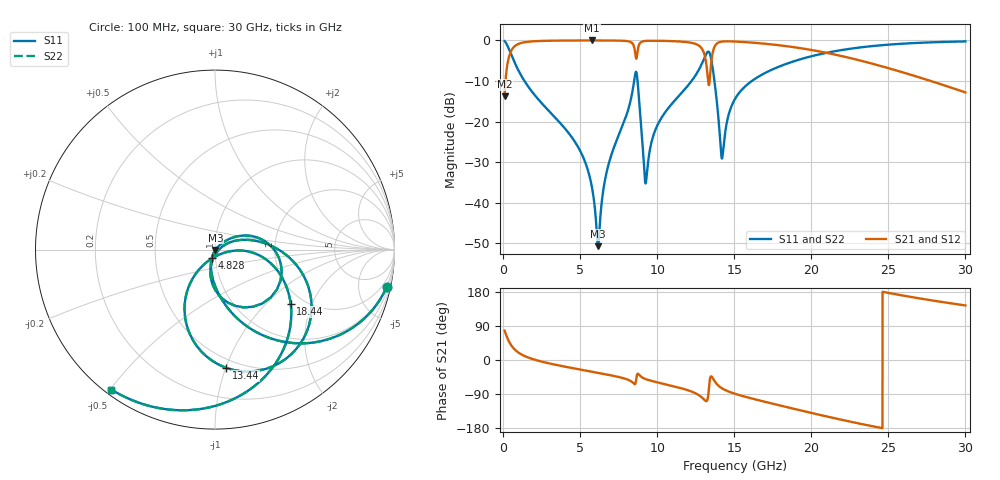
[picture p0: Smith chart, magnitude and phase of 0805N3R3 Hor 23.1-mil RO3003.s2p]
# GHz S MA R 50
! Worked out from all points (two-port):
!   3201 points, 100 MHz to 30 GHz, reference 50 ohm
!   highest |S21| = -0.03 dB at 5.772 GHz (marker M1); lowest = -13.8 dB at 100 MHz (marker M2)
!   |S21| within 3 dB of the highest: 473.9 MHz to 8.572 GHz (8.098 GHz wide, 179 % of centre); 13.6 GHz to 20.93 GHz (7.327 GHz wide, 42.4 % of centre)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
!   lowest |S11| = -50.7 dB at 6.164 GHz (marker M3), VSWR 1.01, Z = 50.2 - j0.164 ohm
!   |S11| at or under -10 dB: 1.388 GHz to 8.504 GHz (7.116 GHz wide, 144 % of centre); 8.726 GHz to 12.23 GHz (3.507 GHz wide, 33.5 % of centre); 13.72 GHz to 16.14 GHz (2.428 GHz wide, 16.3 % of centre)
!   |S22| runs from -50.7 to -0.2 dB; largest |S21 - S12| = 0
!   S11 on the Smith chart (normalised r, x): 100 MHz: 0.92, -9.11; 4.828 GHz: 0.96, -0.09; 13.44 GHz: 0.43, -1.00; 18.44 GHz: 1.72, -1.42; 30 GHz: 0.02, -0.50
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0.1  0.9786 -12.4  0.2053 77.6  0.2053 77.6  0.9786 -12.4
0.4830937  0.701 -48.2  0.7126 41.8  0.7126 41.8  0.701 -48.2
1.258625  0.3467 -76.6  0.9369 13.2  0.9369 13.2  0.3467 -76.6
4.827937  0.05005 -111.3  0.9963 -23.9  0.9963 -23.9  0.05005 -111.3
5.089563  0.04037 -112.5  0.9966 -25.8  0.9966 -25.8  0.04037 -112.5
5.771656  0.01535 -110.9  0.997 -31.0  0.997 -31.0  0.01535 -110.9
6.164094  0.00292 -33.9  0.9969 -33.9  0.9969 -33.9  0.00292 -33.9
6.771438  0.02619 43.7  0.9959 -38.6  0.9959 -38.6  0.02619 43.7
8.574781  0.3843 -15.4  0.6996 -63.1  0.6996 -63.1  0.3843 -15.4
8.752313  0.2765 -81.4  0.7853 -36.2  0.7853 -36.2  0.2765 -81.4
9.247531  0.01728 -37.5  0.9828 -50.3  0.9828 -50.3  0.01728 -37.5
10.06978  0.09462 25.8  0.9877 -59.6  0.9877 -59.6  0.09462 25.8
12.30294  0.3296 2.4  0.9255 -84.4  0.9255 -84.4  0.3296 2.4
13.05978  0.6046 -27.6  0.6755 -105.1  0.6755 -105.1  0.6046 -27.6
13.44288  0.6611 -84.7  0.3925 -46.6  0.3925 -46.6  0.6611 -84.7
13.68581  0.3498 -118.9  0.803 -53.3  0.803 -53.3  0.3498 -118.9
14.19972  0.03501 -66.4  0.9649 -74.5  0.9649 -74.5  0.03501 -66.4
15.05  0.1898 -3.4  0.9671 -89.1  0.9671 -89.1  0.1898 -3.4
18.44178  0.5185 -35.6  0.8457 -124.7  0.8457 -124.7  0.5185 -35.6
20.03956  0.6392 -50.8  0.7595 -140.0  0.7595 -140.0  0.6392 -50.8
25.01978  0.8857 -93.6  0.4539 176.9  0.4539 176.9  0.8857 -93.6
30  0.9704 -126.5  0.2287 144.0  0.2287 144.0  0.9704 -126.5
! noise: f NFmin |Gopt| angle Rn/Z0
0.1  0.0009065  0.933  1.237  0.003009
3.417  0.005982  0.6903  19.46  0.003655
6.743  0.0115  0.6888  36.91  0.006486
10.06  0.02044  0.7388  53.9  0.01252
13.39  0.3986  0.9803  70.43  3.089
16.7  0.02942  0.7208  84.48  0.01169
20.03  0.03418  0.7229  97.62  0.01097
23.35  0.04377  0.755  110.4  0.01224
26.67  0.05861  0.7981  123  0.01425
30  0.08237  0.8458  135.7  0.01679
